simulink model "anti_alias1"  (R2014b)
settings: Solver=ode45  StartTime=0.0  StopTime=5  MaxStep=1e-4  RelTol=1e-3
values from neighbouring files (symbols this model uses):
  ampl1 = 1    [anti_alias_1.m]    (also in anti_alias_2.m; anti_alias_3.m; ad_test_2.m = 0.0001; ad_test_3.m = 0.0001)
  ampl2 = 1/3    (= 0.333333333333)    [anti_alias_1.m]    (also in anti_alias_2.m; anti_alias_3.m; ad_test_2.m = 1e-05; ad_test_3.m = 1e-05)
  ampl3 = 1/5    (= 0.2)    [anti_alias_1.m]    (also in anti_alias_2.m; anti_alias_3.m; fourier_reihe1.m = 6; fourier_reihe2.m = 6)
  ampl4 = 1    [anti_alias_1.m]    (also in anti_alias_2.m; anti_alias_3.m)
  f1 = 50    [anti_alias_1.m]    (also in anti_alias_2.m; anti_alias_3.m; modal_analyse_1.m = imag(lambda(1))/(2*pi),; uebertragung_mechanik_1.m = imag(lambda(1))/(2*pi),)
  f2 = 150    [anti_alias_1.m]    (also in anti_alias_2.m; anti_alias_3.m; modal_analyse_1.m = imag(lambda(3))/(2*pi),; uebertragung_mechanik_1.m = imag(lambda(3))/(2*pi),)
  f3 = 250    [anti_alias_1.m]    (also in anti_alias_2.m; anti_alias_3.m; fourier_reihe1.m = ',num2str(f3),' Hz )']; fourier_reihe2.m = 2300)
  f4 = 1200    [anti_alias_1.m]    (also in anti_alias_2.m; anti_alias_3.m)
  fs = 1000    [anti_alias_1.m]    (also in anti_alias_2.m; anti_alias_3.m; abtast_rate_1.m = 4000; ad_test_12.m = ',     num2str(fs),')
  fst = fs/2    (= 500)    [anti_alias_1.m]
  nfft = 2048    [anti_alias_1.m]    (also in anti_alias_2.m; anti_alias_3.m; freqgang_1.m = 512; impuls_antwort_1.m = 128)
  nord = 6    [analog_filter_3.m]    (also in analog_filter_4.m; analog_filter_5.m; anti_alias_1.m; anti_alias_2.m)
  w = sum(hann(nfft).^2)/nfft    [anti_alias_1.m]    (also in anti_alias_2.m; anti_alias_3.m; freqgang_1.m = (0:nfft-1)/nfft; uebertragung_elektrisch_1.m = rad/s)
undefined symbols (not defined in the file or in its folder): get
libraries: dsparch4 x1, dspspect3 x1, dspsnks4 x1, dspsigops x1

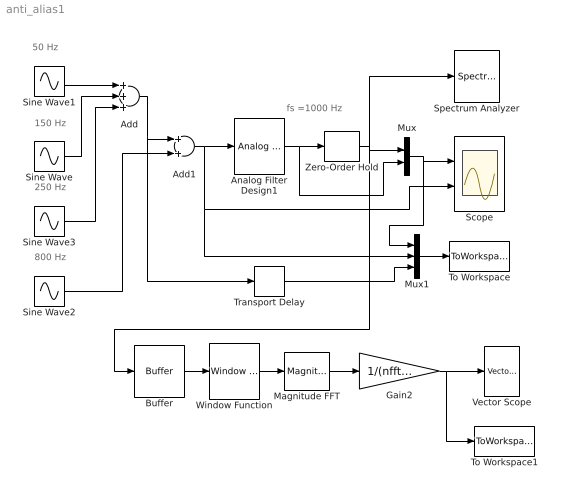
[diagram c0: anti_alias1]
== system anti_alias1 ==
  note: 250 Hz
  note: 800 Hz
  note: 50 Hz
  note: 150 Hz
  note: fs =1000 Hz
  Add : Sum  Inputs=+++
  Add1 : Sum
  Analog Filter Design1 : dsparch4/Analog Filter Design  method=Chebyshev II  filttype=Lowpass  N=nord  Wlo=2*pi*fst  Whi=80  Rp=2  Rs=delta_s
  Buffer : Buffer  N=nfft  TreatMby1Signals=One channel
  Gain2 : Gain  Gain=1/(nfft^2*w)
  Magnitude FFT : dspspect3/Magnitude FFT  mag_or_magsq=Magnitude squared  FFTImplementation=Auto  fftLenInherit=off  fftsize=nfft  WrapInput=on
  Mux : Mux  Inputs=2
  Mux1 : Mux  Inputs=3
  Scope : Scope  NumInputPorts=2
  Sine Wave : Sin  Amplitude=ampl2  Frequency=2*pi*f2  SampleTime=0
  Sine Wave1 : Sin  Amplitude=ampl1  Frequency=2*pi*f1  SampleTime=0
  Sine Wave2 : Sin  Amplitude=ampl4  Frequency=2*pi*f4  SampleTime=0
  Sine Wave3 : Sin  Amplitude=ampl3  Frequency=2*pi*f3  SampleTime=0
  Spectrum Analyzer : SpectrumAnalyzer
  To Workspace : ToWorkspace  VariableName=y  SaveFormat=Timeseries  SampleTime=-1
  To Workspace1 : ToWorkspace  VariableName=Y  SaveFormat=Structure  SampleTime=-1
  Transport Delay : TransportDelay  DelayTime=0.00225
  Vector Scope : dspsnks4/Vector Scope  ScopeProperties=on  Domain=Frequency  HorizSpan=1  DisplayProperties=off  AxisGrid=on  Memory=off  FrameNumber=on  AxisLegend=off  AxisZoom=off  OpenScopeAtSimStart=on  OpenScopeImmediately=off  FigPos=get(0,'defaultfigureposition')  AxisProperties=off  XUnits=Hertz  XRange=[0...Fs]  InheritXIncr=on  XIncr=1  XLabel=Time  XLimit=User-defined  XMin=0  XMax=1000  XStart=0  YUnits=dB  YLabel="Leistung in  dB"  LineProperties=off  XAxisParamsVer=6.9
  Window Function : dspsigops/Window Function  winmode=Apply window to input  wintype=Hanning  sampmode=Continuous  samptime=1  N=64  Rs=50  beta=10  winsamp=Symmetric  UserWindow=hamming  OptParams=off  UserParams={'symmetric'}  RowConvenienceOn=on  dataType=double  isSigned=on  wordLen=16  udDataType=sfix(16)  fracBitsMode=Best precision  numFracBits=15  roundingMode=Floor  overflowMode=off  numSidelobes=4  sidelobeLevel=-30
  Zero-Order Hold : ZeroOrderHold  SampleTime=1/fs
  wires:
  Sine Wave2/1 -> Add1/2
  Add1/1 -> Analog Filter Design1/1, Mux1/2, Scope/2
  Analog Filter Design1/1 -> Mux/2, Zero-Order Hold/1
  Mux/1 -> Mux1/1, Scope/1
  Mux1/1 -> To Workspace/1
  Zero-Order Hold/1 -> Buffer/1, Spectrum Analyzer/1, Mux/1
  Buffer/1 -> Window Function/1
  Magnitude FFT/1 -> Gain2/1
  Gain2/1 -> To Workspace1/1, Vector Scope/1
  Sine Wave1/1 -> Add/1
  Sine Wave/1 -> Add/2
  Window Function/1 -> Magnitude FFT/1
  Add/1 -> Transport Delay/1, Add1/1
  Sine Wave3/1 -> Add/3
  Transport Delay/1 -> Mux1/3
